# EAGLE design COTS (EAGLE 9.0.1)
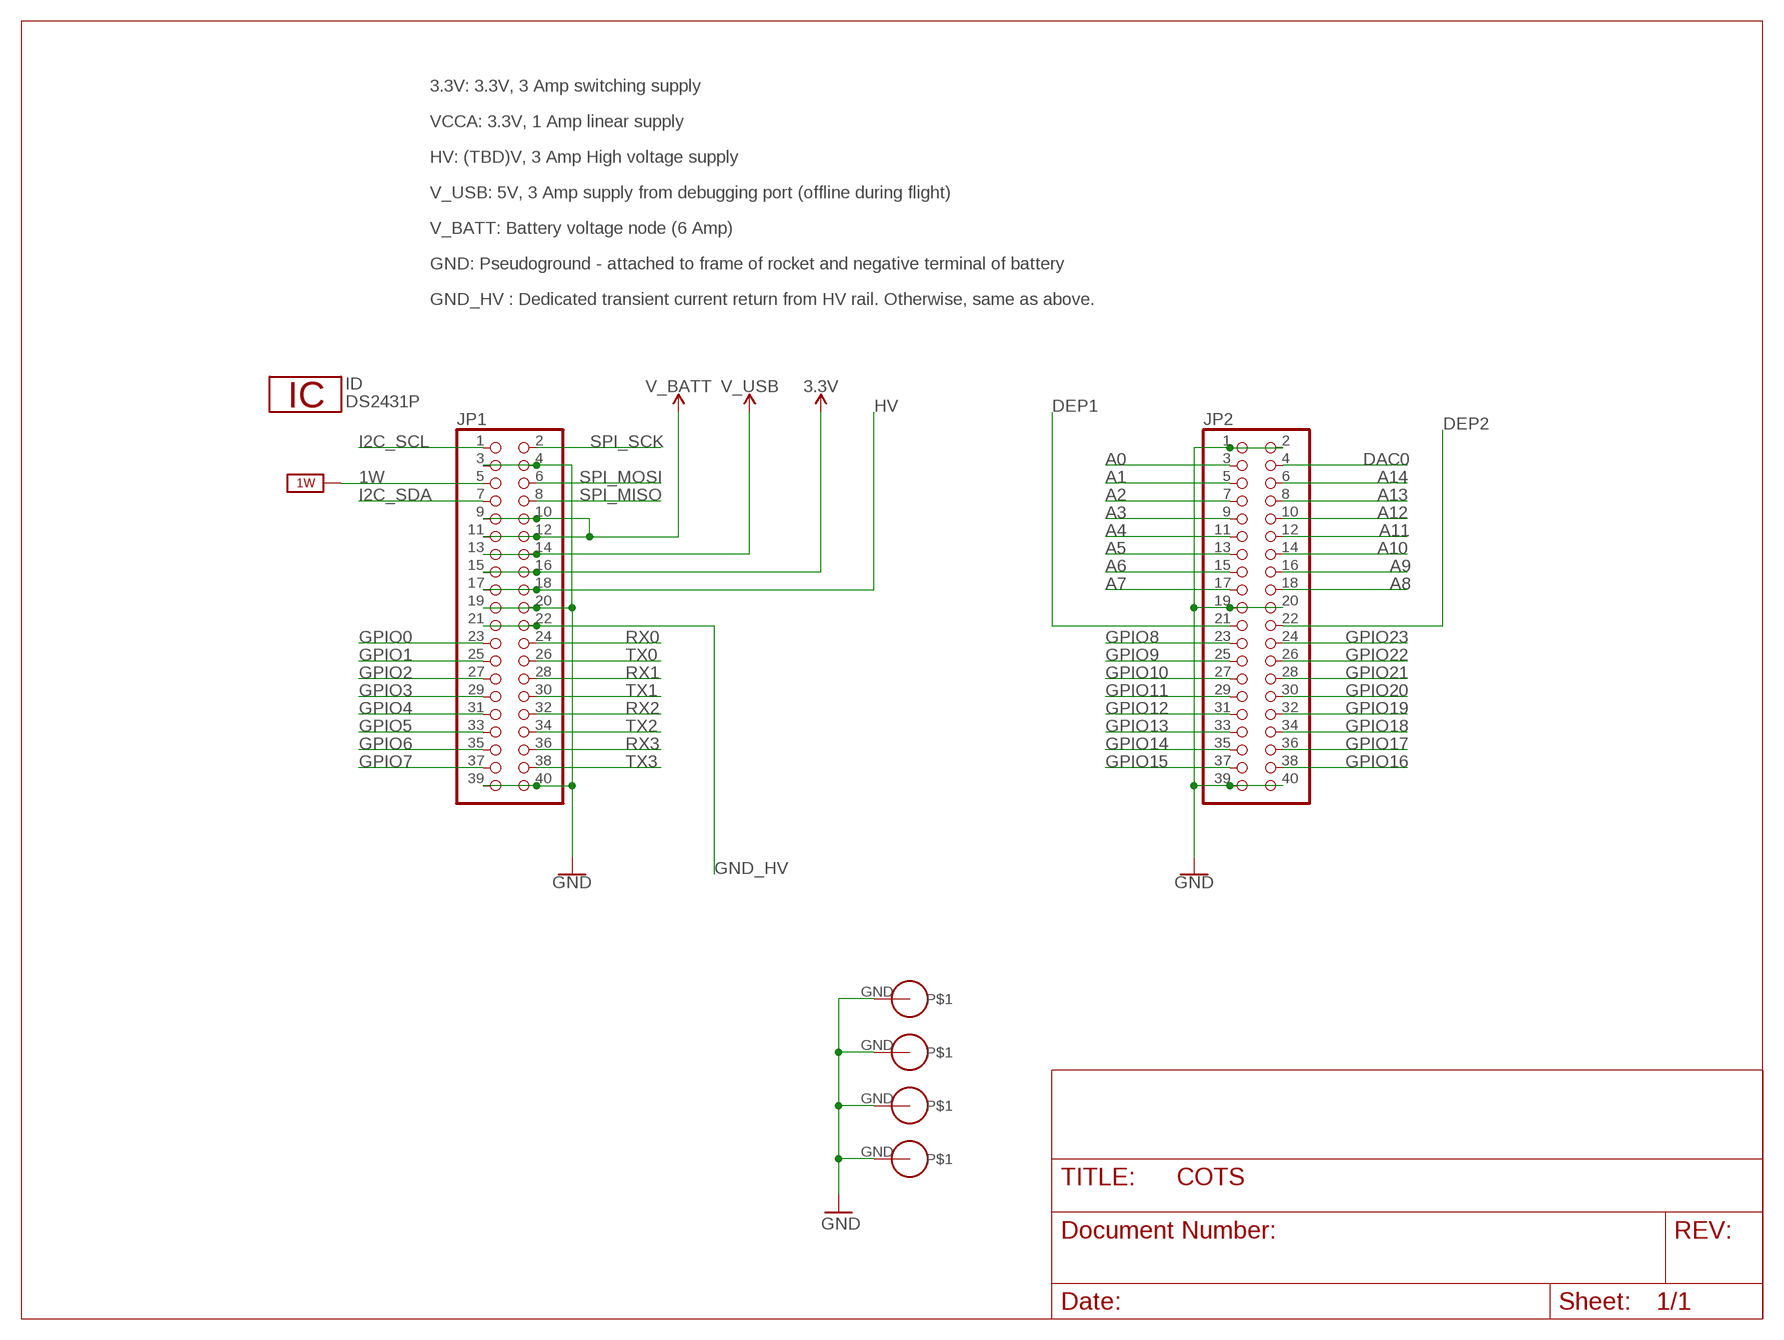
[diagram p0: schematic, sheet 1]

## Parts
ID  DS2431P  [TSOC6]
JP1  PINHD-2X20  [2X20]
JP2  PINHD-2X20  [2X20]
U$1  PS/104-MOUNTING-HOLE  [PC/104-MOUNTING-HOLE]
U$2  PS/104-MOUNTING-HOLE  [PC/104-MOUNTING-HOLE]
U$3  PS/104-MOUNTING-HOLE  [PC/104-MOUNTING-HOLE]
U$4  PS/104-MOUNTING-HOLE  [PC/104-MOUNTING-HOLE]

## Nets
1W: JP1.5 ; supply symbol labelled 1W_SUP
3.3V: JP1.15 JP1.16
A0: JP2.3
A1: JP2.5
A2: JP2.7
A3: JP2.9
A4: JP2.11
A5: JP2.13
A6: JP2.15
A7: JP2.17
A8: JP2.18
A9: JP2.16
A10: JP2.14
A11: JP2.12
A12: JP2.10
A13: JP2.8
A14: JP2.6
DAC0: JP2.4
DEP1: JP2.21
DEP2: JP2.22
GND: JP1.3 JP1.4 JP1.19 JP1.20 JP1.39 JP1.40 JP2.1 JP2.2 JP2.19 JP2.20 JP2.39 JP2.40 U$1.GND U$2.GND U$3.GND U$4.GND
GND_HV: JP1.21 JP1.22
GPIO0: JP1.23
GPIO8: JP2.23
GPIO9: JP2.25
GPIO10: JP2.27
GPIO11: JP2.29
GPIO12: JP2.31
GPIO13: JP2.33
GPIO14: JP2.35
GPIO15: JP2.37
GPIO16: JP2.38
GPIO17: JP2.36
GPIO18: JP2.34
GPIO19: JP2.32
GPIO20: JP2.30
GPIO21: JP2.28
GPIO22: JP2.26
GPIO23: JP2.24
HV: JP1.17 JP1.18
I2C_SCL: JP1.1
I2C_SDA: JP1.7
RX0: JP1.24
RX1: JP1.28
RX2: JP1.32
RX3: JP1.36
SPI_MISO: JP1.8
SPI_MOSI: JP1.6
SPI_SCK: JP1.2
TX0: JP1.26
TX1: JP1.30
TX2: JP1.34
TX3: JP1.38
V_BATT: JP1.9 JP1.10 JP1.11 JP1.12
V_USB: JP1.13 JP1.14
Unconnected: JP1.25 JP1.27 JP1.29 JP1.31 JP1.33 JP1.35 JP1.37

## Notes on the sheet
- 3.3V: 3.3V, 3 Amp switching supply
- VCCA: 3.3V, 1 Amp linear supply
- HV: (TBD)V, 3 Amp High voltage supply
- V_USB: 5V, 3 Amp supply from debugging port (offline during flight)
- V_BATT: Battery voltage node (6 Amp)
- GND: Pseudoground - attached to frame of rocket and negative terminal of battery
- GND_HV : Dedicated transient current return from HV rail. Otherwise, same as above.

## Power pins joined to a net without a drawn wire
1W: ID.2(1W)
GND: ID.1(GND)

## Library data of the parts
ID = 1wire:DS2431: 1024-Bit EEPROM
JP1 JP2 = pinhead:PINHD-2X20: PIN HEADER
U$1-U$4 = CU inSpace 2019 Parts:PS/104-MOUNTING-HOLE: Mounting hole for PC/104 board.

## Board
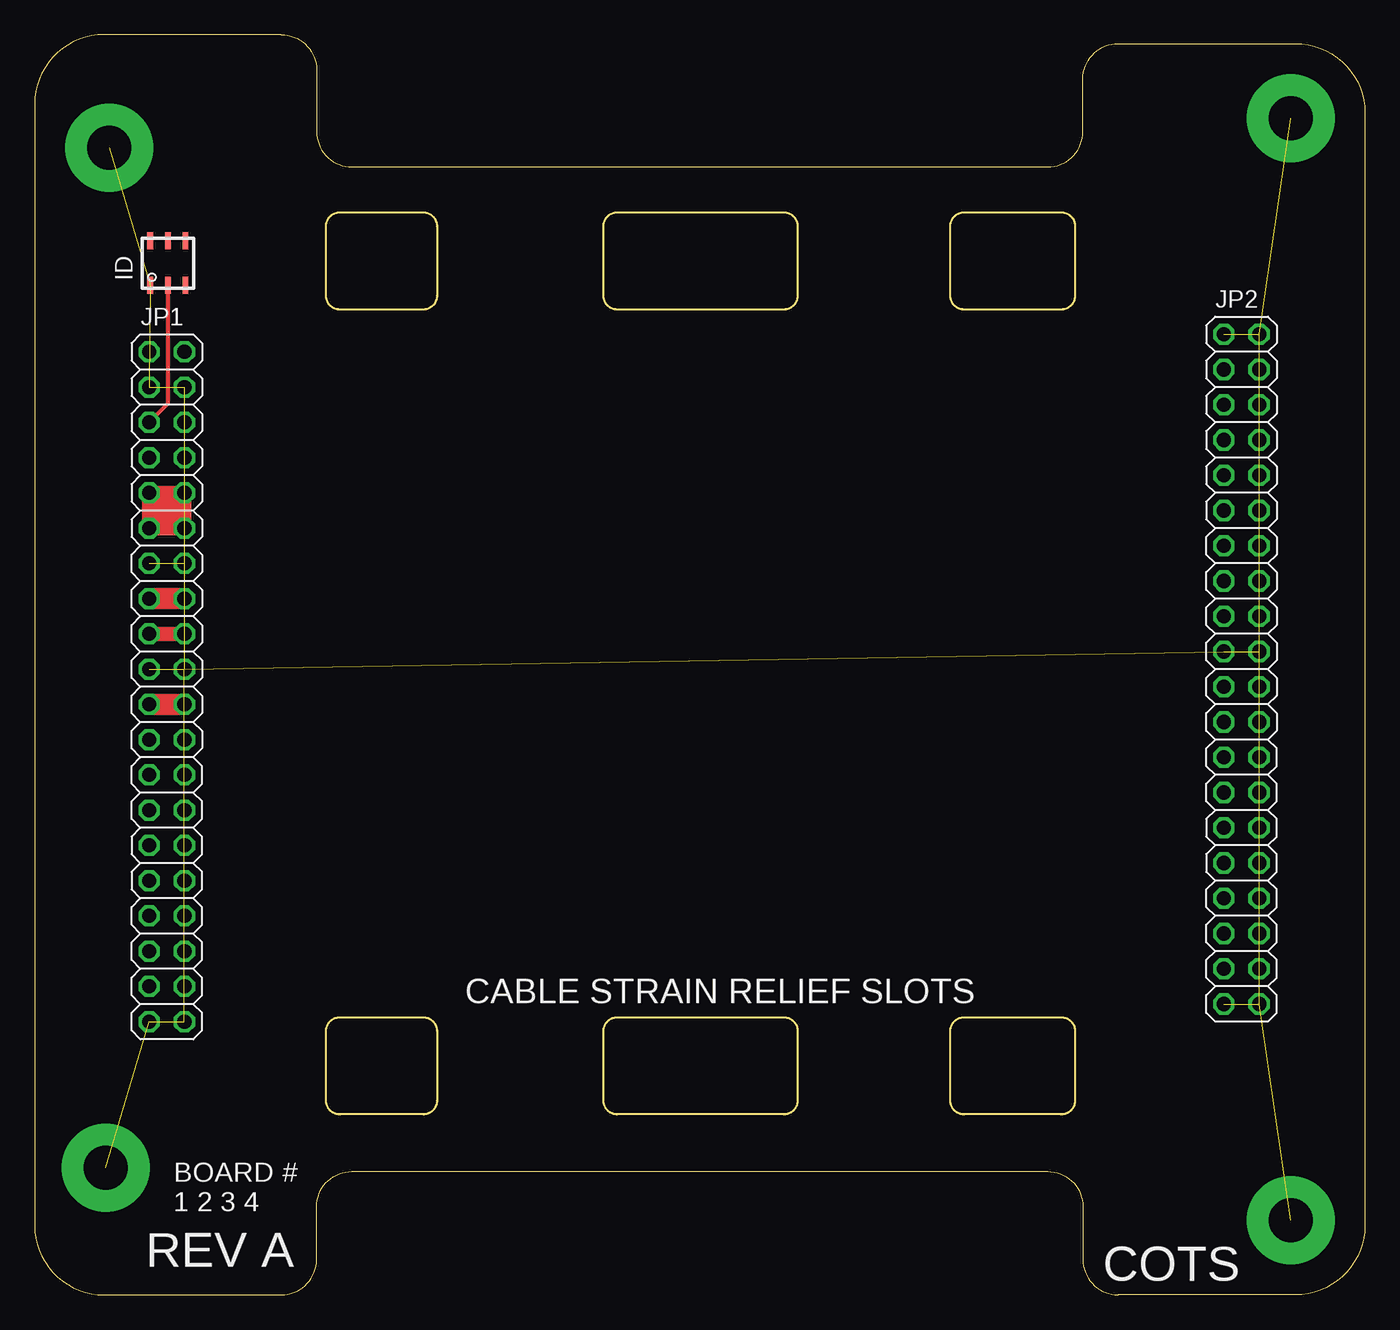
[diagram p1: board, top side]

Size 95.89 x 90.81 mm. Coordinates in mm from the lower left corner, seen from the top.
Outline: 72 segments
Copper layers (1*16): Top 0.035mm / dielectric 1.5mm / Bottom 0.035mm
Design rules "default": minimum track width 6mil, minimum drill 0.35mm, track to track 6mil, track to pad 6mil, pad to pad 6mil, via to via 6mil, smd to smd 6mil, copper to edge 40mil, drill to drill 6mil, minimum pad ring 10mil, minimum via ring 8mil, stop-mask expansion 4mil, vias tented up to drill 0mil, thermal gap 10mil

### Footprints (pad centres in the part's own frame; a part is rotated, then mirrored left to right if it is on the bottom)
TSOC6 = smd 0.406 x 1.219: 1 -1.27,-1.6; 2 0,-1.6; 3 1.27,-1.6; 4 1.27,1.6; 5 0,1.6; 6 -1.27,1.6
2X20 = drill 1.016 octagon: 1 -24.13,-1.27; 2 -24.13,1.27; 3 -21.59,-1.27; 4 -21.59,1.27; 5 -19.05,-1.27; 6 -19.05,1.27; 7 -16.51,-1.27; 8 -16.51,1.27; 9 -13.97,-1.27; 10 -13.97,1.27; 11 -11.43,-1.27; 12 -11.43,1.27; 13 -8.89,-1.27; 14 -8.89,1.27; 15 -6.35,-1.27; 16 -6.35,1.27; 17 -3.81,-1.27; 18 -3.81,1.27; 19 -1.27,-1.27; 20 -1.27,1.27; 21 1.27,-1.27; 22 1.27,1.27; 23 3.81,-1.27; 24 3.81,1.27; 25 6.35,-1.27; 26 6.35,1.27; 27 8.89,-1.27; 28 8.89,1.27; 29 11.43,-1.27; 30 11.43,1.27; 31 13.97,-1.27; 32 13.97,1.27; 33 16.51,-1.27; 34 16.51,1.27; 35 19.05,-1.27; 36 19.05,1.27; 37 21.59,-1.27; 38 21.59,1.27; 39 24.13,-1.27; 40 24.13,1.27
PC/104-MOUNTING-HOLE = drill 3.175 pad 6.35: GND 0,0

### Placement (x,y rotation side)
ID  9.6,74.35 0 top
JP1  9.53,43.81 270 top
JP2  87,45.09 270 top
U$1  5.36,82.65 0 top
U$2  90.55,84.79 0 top
U$3  5.13,9.17 0 top
U$4  90.55,5.36 0 top

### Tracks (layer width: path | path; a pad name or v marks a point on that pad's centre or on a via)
1W
  Top 0.305: ID.2 9.6,64.21 JP1.5
3.3V
  Top 1.016: JP1.16 10.79,50.13
  Top 1.5: JP1.16 JP1.15
GND  (16 unrouted)
GND_HV
  Top 1.5: JP1.21 JP1.22
HV
  Top 1.016: JP1.17 JP1.18
V_BATT
  Top 1.016: 9,55.24 JP1.11 JP1.9 | 9,55.24 10,55.24 | 10,55.24 JP1.12 JP1.10 10,57.78 | JP1.9 10,57.78 | JP1.9 9,57.78 9,55.24 | 10,55.24 10,57.78
V_USB  (1 unrouted)

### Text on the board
tPlace: CABLE STRAIN RELIEF SLOTS | BOARD # / 1 2 3 4 | REV A | COTS

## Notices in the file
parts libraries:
SparkFun-PowerSymbols: Licensing: Creative Commons ShareAlike 4.0 International - https://creativecommons.org/licenses/by-sa/4.0
